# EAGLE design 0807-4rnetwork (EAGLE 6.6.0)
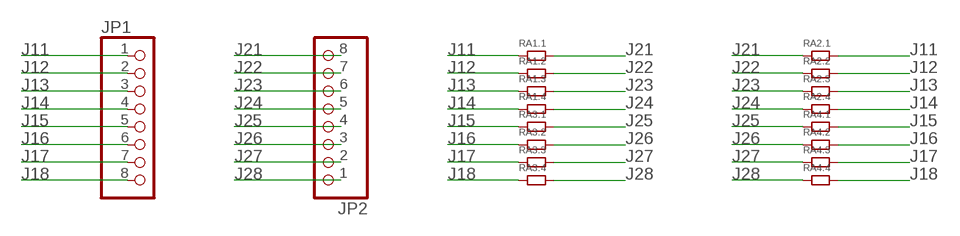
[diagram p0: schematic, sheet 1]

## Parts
JP1  PINHD-1X8CLEANBIG  [1X08-CLEANBIG]
JP2  PINHD-1X8CLEANBIG  [1X08-CLEANBIG]
RA1  RA-4.0603  [0603.4.C]
RA2  RA-4.0402  [0402.4.C]
RA3  RA-4.0603  [0603.4.C]
RA4  RA-4.0402  [0402.4.C]

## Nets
J11: JP1.1 RA1.1 RA2.2
J12: JP1.2 RA1.3 RA2.4
J13: JP1.3 RA1.5 RA2.6
J14: JP1.4 RA1.7 RA2.8
J15: JP1.5 RA3.1 RA4.2
J16: JP1.6 RA3.3 RA4.4
J17: JP1.7 RA3.5 RA4.6
J18: JP1.8 RA3.7 RA4.8
J21: JP2.8 RA1.2 RA2.1
J22: JP2.7 RA1.4 RA2.3
J23: JP2.6 RA1.6 RA2.5
J24: JP2.5 RA1.8 RA2.7
J25: JP2.4 RA3.2 RA4.1
J26: JP2.3 RA3.4 RA4.3
J27: JP2.2 RA3.6 RA4.5
J28: JP2.1 RA3.8 RA4.7

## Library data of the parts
JP1 JP2 = adafruit:PINHD-1X8: PIN HEADER
RA1-RA4 = resistorarray:RA-4: Dimentions sources from here: http://www.ctscorp.com/components/Datasheets/CTSChipArrayDs.pdf

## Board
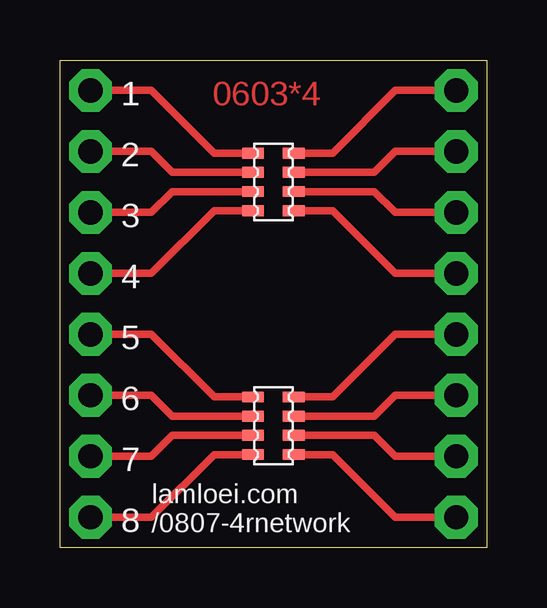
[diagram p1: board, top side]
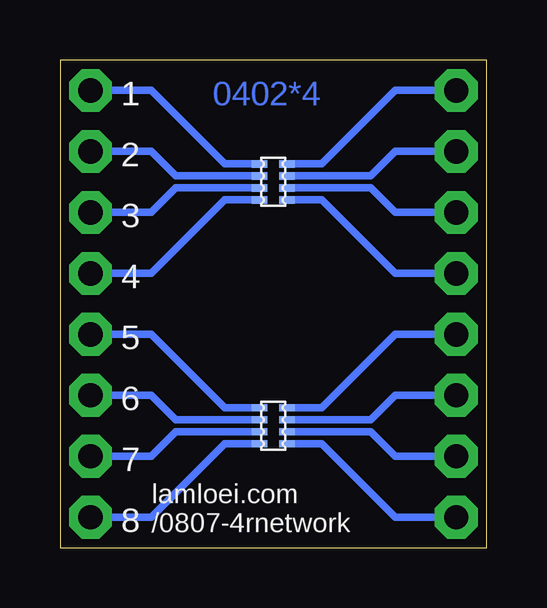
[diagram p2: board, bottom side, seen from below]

Size 17.78 x 20.32 mm. Coordinates in mm from the lower left corner, seen from the top.
Outline: 0,0 0,20.32 17.78,20.32 17.78,0 0,0
Copper layers (1*16): Top 0.0356mm / dielectric 1.5011mm / Bottom 0.0356mm
Design rules "oshpark-2layer": minimum track width 6mil, minimum drill 13mil, track to track 6mil, track to pad 6mil, pad to pad 6mil, via to via 6mil, smd to smd 6mil, copper to edge 15mil, drill to drill 6mil, minimum pad ring 7mil, minimum via ring 7mil, stop-mask expansion 4mil, vias tented up to drill 0mil, thermal gap 10mil

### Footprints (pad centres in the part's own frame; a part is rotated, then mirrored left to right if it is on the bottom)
1X08-CLEANBIG = drill 1.016 pad 1.778 octagon: 1 -8.89,0; 2 -6.35,0; 3 -3.81,0; 4 -1.27,0; 5 1.27,0; 6 3.81,0; 7 6.35,0; 8 8.89,0
0603.4.C = smd 0.45 x 0.9: 1 -1.2,-0.85; 2 -1.2,0.85; 3 -0.4,-0.85; 4 -0.4,0.85; 5 0.4,-0.85; 6 0.4,0.85; 7 1.2,-0.85; 8 1.2,0.85
0402.4.C = smd 0.3 x 0.65: 1 -0.75,-0.575; 2 -0.75,0.575; 3 -0.25,-0.575; 4 -0.25,0.575; 5 0.25,-0.575; 6 0.25,0.575; 7 0.75,-0.575; 8 0.75,0.575

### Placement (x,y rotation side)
JP1  1.27,10.16 270 top
JP2  16.51,10.16 90 top
RA1  8.89,15.24 270 top
RA2  8.89,15.24 270 bottom
RA3  8.89,5.08 270 top
RA4  8.89,5.08 270 bottom

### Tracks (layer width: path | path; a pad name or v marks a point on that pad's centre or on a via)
J11
  Top 0.305: RA1.1 6.42,16.44 3.81,19.05 JP1.1
  Bottom 0.305: RA2.2 6.87,15.99 3.81,19.05 JP1.1
J12
  Top 0.305: RA1.3 4.68,15.64 3.81,16.51 JP1.2
  Bottom 0.305: RA2.4 4.83,15.49 3.81,16.51 JP1.2
J13
  Top 0.305: RA1.5 4.68,14.84 3.81,13.97 JP1.3
  Bottom 0.305: RA2.6 4.83,14.99 3.81,13.97 JP1.3
J14
  Top 0.305: RA1.7 6.42,14.04 3.81,11.43 JP1.4
  Bottom 0.305: RA2.8 6.87,14.49 3.81,11.43 JP1.4
J15
  Top 0.305: RA3.1 6.42,6.28 3.81,8.89 JP1.5
  Bottom 0.305: RA4.2 6.87,5.83 3.81,8.89 JP1.5
J16
  Top 0.305: RA3.3 4.68,5.48 3.81,6.35 JP1.6
  Bottom 0.305: RA4.4 4.83,5.33 3.81,6.35 JP1.6
J17
  Top 0.305: RA3.5 4.68,4.68 3.81,3.81 JP1.7
  Bottom 0.305: RA4.6 4.83,4.83 3.81,3.81 JP1.7
J18
  Top 0.305: RA3.7 6.42,3.88 3.81,1.27 JP1.8
  Bottom 0.305: RA4.8 6.87,4.33 3.81,1.27 JP1.8
J21
  Top 0.305: RA1.2 11.36,16.44 13.97,19.05 JP2.8
  Bottom 0.305: RA2.1 10.91,15.99 13.97,19.05 JP2.8
J22
  Top 0.305: RA1.4 13.1,15.64 13.97,16.51 JP2.7
  Bottom 0.305: RA2.3 12.95,15.49 13.97,16.51 JP2.7
J23
  Top 0.305: RA1.6 13.1,14.84 13.97,13.97 JP2.6
  Bottom 0.305: RA2.5 12.95,14.99 13.97,13.97 JP2.6
J24
  Top 0.305: RA1.8 11.36,14.04 13.97,11.43 JP2.5
  Bottom 0.305: RA2.7 10.91,14.49 13.97,11.43 JP2.5
J25
  Top 0.305: RA3.2 11.36,6.28 13.97,8.89 JP2.4
  Bottom 0.305: RA4.1 10.91,5.83 13.97,8.89 JP2.4
J26
  Top 0.305: RA3.4 13.1,5.48 13.97,6.35 JP2.3
  Bottom 0.305: RA4.3 12.95,5.33 13.97,6.35 JP2.3
J27
  Top 0.305: RA3.6 13.1,4.68 13.97,3.81 JP2.2
  Bottom 0.305: RA4.5 12.95,4.83 13.97,3.81 JP2.2
J28
  Top 0.305: RA3.8 11.36,3.88 13.97,1.27 JP2.1
  Bottom 0.305: RA4.7 10.91,4.33 13.97,1.27 JP2.1

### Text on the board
Top: 0603*4
Bottom: 0402*4
tPlace: 1 | 2 | 3 | 4 | 5 | 6 | 7 | 8 | lamloei.com / /0807-4rnetwork
bPlace: 1 | 2 | 3 | 4 | 5 | 6 | 7 | lamloei.com / /0807-4rnetwork | 8
tStop: 0603*4
bStop: 0402*4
